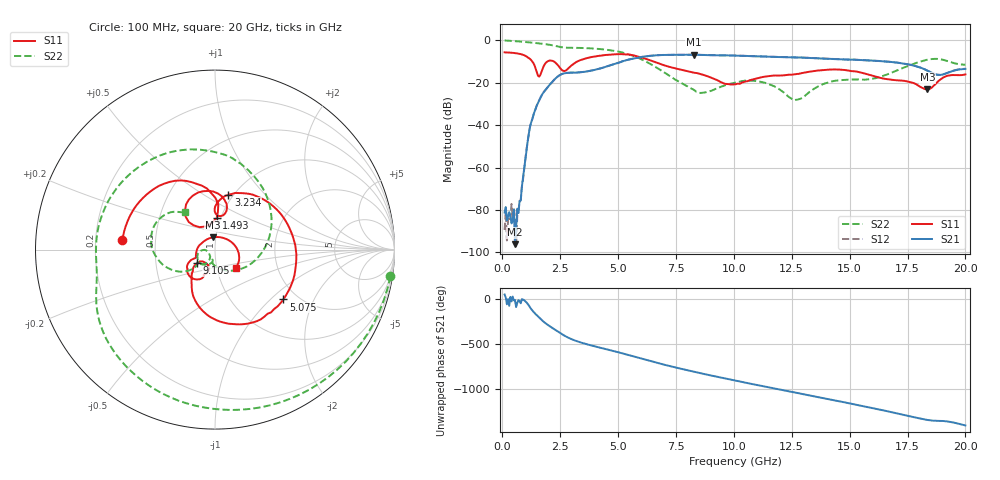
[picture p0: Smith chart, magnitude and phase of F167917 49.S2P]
!  2-Port S-parameters saved by WinCal
! VAR MeasName=S-Parameters (CALIBRATED_DATA) read from VNA (N5242A)
! VAR MeasDate=2016-11-22 9:02:18
! VAR NAME=F167917 49
! VAR FILENAME=F167917 49.S2P
! VAR DATE=2016-11-22 9:02:18
! VAR PHYS_PORTS=1,2
# Hz S DB R 50
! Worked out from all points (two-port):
!   401 points, 100 MHz to 20 GHz, reference 50 ohm
!   highest |S21| = -6.81 dB at 8.259 GHz (marker M1); lowest = -96.1 dB at 547.8 MHz (marker M2)
!   |S21| within 3 dB of the highest: 5.23 GHz to 16.31 GHz (11.08 GHz wide, 103 % of centre)
!   lowest |S11| = -23.2 dB at 18.36 GHz (marker M3), VSWR 1.15, Z = 48.4 + j6.65 ohm
!   |S11| at or under -10 dB: 1.291 GHz to 1.949 GHz (657.8 MHz wide, 40.6 % of centre); 2.224 GHz to 3.242 GHz (1.018 GHz wide, 37.3 % of centre); 6.53 GHz to end of sweep
!   |S22| runs from -28.3 to -0.1 dB; largest |S21 - S12| = 0.0041
!   S11 on the Smith chart (normalised r, x): 100 MHz: 0.32, +0.05; 1.493 GHz: 0.96, +0.35; 3.234 GHz: 0.95, +0.64; 5.075 GHz: 1.69, -1.21; 9.105 GHz: 0.81, -0.12; 20 GHz: 1.24, -0.26
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1e8  -5.71 174.2  -81.17 53.8  -89.36 50.6  -0.10 -8.7
5.4775e8  -6.05 147.4  -96.07 -6.6  -83.10 -96.5  -0.40 -44.6
7.4675e8  -6.40 134.5  -75.84 -18.9  -75.69 6.1  -0.58 -59.6
1.14475e9  -8.40 105.5  -44.11 -67.1  -44.15 -67.2  -0.99 -87.6
1.493e9  -15.13 87.1  -30.65 -178.0  -30.65 -177.7  -1.37 -109.7
1.84125e9  -11.20 127.4  -23.71 98.7  -23.69 98.7  -1.82 -129.9
2.3885e9  -11.57 75.9  -17.12 2.6  -17.11 2.6  -2.91 -157.7
3.23425e9  -10.03 76.3  -15.17 -107.9  -15.16 -107.9  -3.58 171.4
3.43325e9  -9.15 64.3  -15.02 -124.6  -15.01 -124.6  -3.64 163.2
5.075e9  -6.53 -36.1  -10.42 125.4  -10.42 125.4  -5.47 85.0
5.92075e9  -7.81 -84.2  -8.07 65.0  -8.03 65.1  -8.55 33.4
6.7665e9  -10.94 -115.5  -7.02 6.0  -7.00 6.0  -13.58 -23.9
8.259e9  -15.23 -135.8  -6.81 -86.4  -6.80 -86.4  -23.31 -105.5
9.10475e9  -17.98 -143.0  -7.07 -134.3  -7.04 -134.5  -23.43 -101.8
1.005e10  -20.79 -120.2  -7.22 174.5  -7.22 174.6  -20.01 -122.8
1.1642e10  -16.72 -111.7  -7.78 91.5  -7.75 91.5  -21.20 -172.5
1.2637e10  -16.09 -113.1  -8.07 40.8  -8.06 40.7  -28.22 -152.8
1.338325e10  -14.65 -117.3  -8.39 1.8  -8.34 2.0  -23.44 -118.8
1.51245e10  -14.57 -144.9  -9.14 -86.7  -9.10 -87.0  -18.49 -142.7
1.67165e10  -18.49 -156.6  -10.12 -173.3  -10.17 -173.4  -15.70 -139.2
1.835825e10  -23.18 99.7  -14.32 94.3  -14.27 94.4  -9.15 180.0
2e10  -16.09 -40.6  -13.51 33.0  -13.43 33.3  -11.53 128.4
